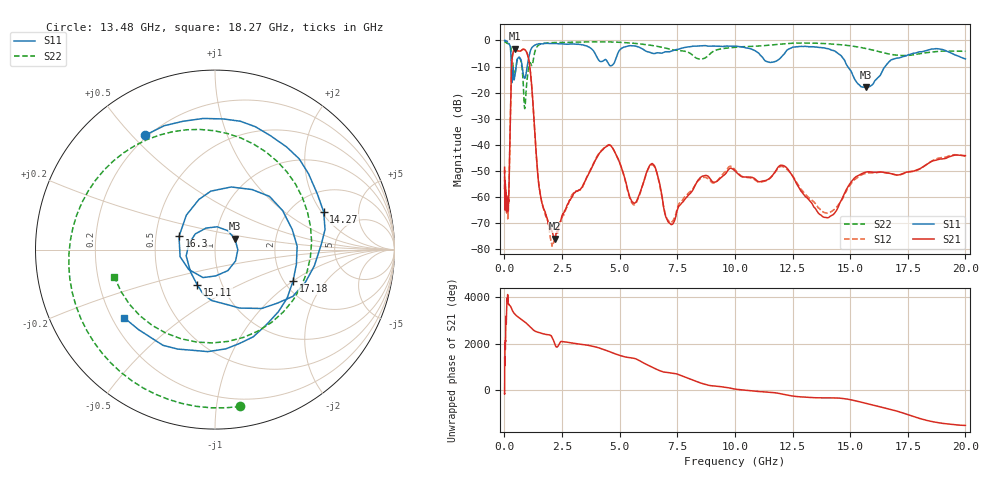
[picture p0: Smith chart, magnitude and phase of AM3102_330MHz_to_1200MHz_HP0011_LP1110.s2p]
! Date/Time: Tue, Sep 11, 2018 5:12 PM
! Network Analyzer: Agilent Technologies E8362B Rev: A.07.50.63
! Sweep from 0.010 to 20.000 GHz, 1601 Points, Sweep Type: LOG
! Power Supply: 4.949 V, 0.001 A
# Hz S DB R 50
!freq MagS11 AngS11 MagS21 AngS21 MagS12 AngS12 MagS22 AngS22
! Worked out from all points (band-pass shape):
!   1601 points, 10 MHz to 20 GHz, reference 50 ohm
!   highest |S21| = -3.19 dB at 475.7 MHz (marker M1); lowest = -75.9 dB at 2.175 GHz (marker M2)
!   |S21| within 3 dB of the highest: 344.5 MHz to 1.028 GHz (683.9 MHz wide, 99.6 % of centre)
!   lowest |S11| = -18.0 dB at 15.7 GHz (marker M3), VSWR 1.29, Z = 61.9 + j7.62 ohm
!   |S11| at or under -10 dB: 298.8 MHz to 505.7 MHz (206.9 MHz wide, 51.4 % of centre); 772 MHz to 988 MHz (216 MHz wide, 24.5 % of centre); 14.89 GHz to 16.52 GHz (1.623 GHz wide, 10.3 % of centre)
!   |S22| runs from -26.1 to -0.3 dB; largest |S21 - S12| = 0.012
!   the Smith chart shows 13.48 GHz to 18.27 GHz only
!   S11 on the Smith chart (normalised r, x): 13.48 GHz: 0.19, +0.55; 14.27 GHz: 2.95, +2.10; 15.11 GHz: 0.76, -0.31; 16.3 GHz: 0.66, +0.10; 17.18 GHz: 2.23, -1.00; 18.27 GHz: 0.25, -0.32
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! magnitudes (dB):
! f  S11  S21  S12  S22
! 10 MHz  0.0  -48.6  -50.6  -0.3
! 35.55 MHz  0.0  -62.0  -59.6  -0.6
! 126.4 MHz  -0.4  -64.1  -64.6  -1.1
! 171.3 MHz  -0.8  -63.3  -66.4  -1.3
! 313.2 MHz  -15.5  -9.9  -9.9  -4.9
! 447.2 MHz  -14.0  -3.3  -3.3  -13.1
! 475.7 MHz  -12.5  -3.2  -3.2  -11.8
! 882.2 MHz  -14.5  -3.5  -3.6  -26.1
! 1.052 GHz  -6.9  -7.1  -7.1  -10.2
! 1.59 GHz  -1.3  -60.5  -60.5  -1.4
! 2.175 GHz  -1.2  -75.9  -76.1  -0.8
! 4.436 GHz  -7.7  -40.5  -40.4  -0.5
! 5.652 GHz  -2.1  -62.3  -62.9  -1.1
! 12.03 GHz  -6.2  -47.8  -48.3  -1.4
! 13.48 GHz  -2.5  -64.2  -62.4  -1.1
! 14.27 GHz  -3.9  -66.6  -65.0  -1.4
! 15.11 GHz  -13.2  -53.5  -54.0  -2.2
! 15.7 GHz  -18.0  -50.4  -50.8  -3.1
! 16.3 GHz  -13.4  -50.4  -50.5  -4.4
! 17.18 GHz  -6.6  -51.4  -51.4  -5.8
! 18.27 GHz  -4.0  -47.7  -47.8  -4.7
! 20 GHz  -7.1  -44.1  -44.4  -4.2
